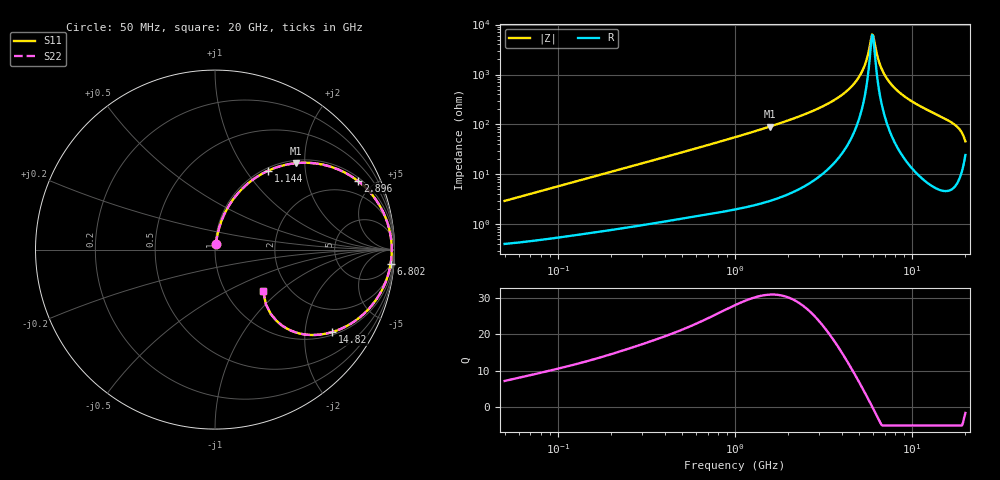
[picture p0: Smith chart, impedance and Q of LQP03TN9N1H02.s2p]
!Murata Part Number: LQP03TN9N1H02
!These Parameters are Measured in Series Mode Connection
!  o--[Z]--o
!Port1  Port2
!  o-------o
!Freq. Start=50[MHz] Stop=20[GHz], 401[Steps]
# Hz S RI R 50
!Freq.(Hz) S11(Real) S11(Imag) S21(Real) S21(Imag) S12(Real) S12(Imag) S22(Real) S22(Imag)
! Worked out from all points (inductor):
!   401 points, 50 MHz to 20 GHz, reference 50 ohm
!   read as one part in series: L = 9.24 nH near 51.52 MHz
!   highest Q = 30.8 at 1.567 GHz (marker M1), where L = 9.18 nH
!   self-resonance near 5.944 GHz
!   S11 on the Smith chart (normalised r, x): 50 MHz: 1.01, +0.06; 1.144 GHz: 1.04, +1.28; 2.896 GHz: 1.17, +4.05; 6.802 GHz: 5, -24; 14.82 GHz: 1.09, -2.78; 20 GHz: 1.49, -0.78
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5e7  0.00489 0.029  0.9951 -0.029  0.9951 -0.029  0.00489 0.029
1.364002e8  0.0121 0.076  0.9879 -0.076  0.9879 -0.076  0.0121 0.076
3.721004e8  0.0502 0.1934  0.9498 -0.1934  0.9498 -0.1934  0.0502 0.1934
1e9  0.2437 0.4118  0.7563 -0.4118  0.7563 -0.4118  0.2437 0.4118
1.144317e9  0.2972 0.4402  0.7028 -0.4402  0.7028 -0.4402  0.2972 0.4402
1.567309e9  0.4516 0.4817  0.5484 -0.4817  0.5484 -0.4817  0.4516 0.4817
2.728004e9  0.7642 0.4054  0.2358 -0.4054  0.2358 -0.4054  0.7642 0.4054
2.896447e9  0.7944 0.3841  0.2056 -0.3841  0.2056 -0.3841  0.7944 0.3841
3.850025e9  0.9117 0.2547  0.0883 -0.2547  0.0883 -0.2547  0.9117 0.2547
4.748272e9  0.9643 0.1381  0.0357 -0.1381  0.0357 -0.1381  0.9643 0.1381
5.352748e9  0.9799 0.0669  0.0201 -0.0669  0.0201 -0.0669  0.9799 0.0669
5.856089e9  0.9846 0.0123  0.0154 -0.0123  0.0154 -0.0123  0.9846 0.0123
5.944466e9  0.9848 0.00311  0.0152 -0.00311  0.0152 -0.00311  0.9848 0.00311
6.125241e9  0.9846 -0.0152  0.0154 0.0152  0.0154 0.0152  0.9846 -0.0152
6.503449e9  0.9822 -0.0518  0.0178 0.0518  0.0178 0.0518  0.9822 -0.0518
6.802353e9  0.9786 -0.0793  0.0214 0.0793  0.0214 0.0793  0.9786 -0.0793
7.442007e9  0.9666 -0.1336  0.0334 0.1336  0.0334 0.1336  0.9666 -0.1336
9.745021e9  0.892 -0.2873  0.108 0.2873  0.108 0.2873  0.892 -0.2873
1.482269e10  0.6537 -0.4591  0.3463 0.4591  0.3463 0.4591  0.6537 -0.4591
1.800918e10  0.4488 -0.4611  0.5512 0.4611  0.5512 0.4611  0.4488 -0.4611
1.88369e10  0.3713 -0.4216  0.6287 0.4216  0.6287 0.4216  0.3713 -0.4216
2e10  0.2685 -0.2286  0.7315 0.2286  0.7315 0.2286  0.2685 -0.2286
